DATA_BLOCK DB 63
VERSION : 0.1


  STRUCT
   Messwert : REAL  := 1.000000e+000;
   Messwert1 : REAL  := 1.500000e+000;
   Messwert2 : REAL  := 2.000000e+000;
   Messwert3 : REAL  := 2.500000e+000;
   Messwert4 : REAL  := 3.000000e+000;
   Messwert5 : REAL  := 3.500000e+000;
   Messwert6 : REAL  := 4.000000e+000;
   Messwert7 : REAL  := 4.500000e+000;
   Messwert8 : REAL  := 5.000000e+000;
   Messwert9 : REAL  := 5.500000e+000;
   Messwert10 : REAL  := 6.000000e+000;
   Messwert11 : REAL  := 6.500000e+000;
   Messwert12 : REAL  := 7.000000e+000;
   Messwert13 : REAL  := 7.500000e+000;
   Messwert14 : REAL  := 8.000000e+000;
   Messwert15 : REAL  := 8.500000e+000;
   Messwert16 : REAL  := 9.000000e+000;
   Messwert17 : REAL  := 9.500000e+000;
   Messwert18 : REAL  := 5.000000e-001;
   Messwert19 : REAL  := 1.000000e-001;
   Messwert20 : REAL  := 1.500000e-001;
   Messwert21 : REAL  := 2.500000e-001;
   Messwert22 : REAL  := 3.500000e-001;
   Messwert23 : REAL  := 4.500000e-001;
   Messwert24 : REAL  := 5.500000e-001;
   Messwert25 : REAL  := 6.500000e-001;
   Messwert26 : REAL  := 7.500000e-001;
   Messwert27 : REAL  := 8.500000e-001;
   Messwert28 : REAL  := 9.500000e-001;
   Messwert29 : REAL  := 2.000000e-001;
  END_STRUCT ;
BEGIN
   Messwert := 1.000000e+000;
   Messwert1 := 1.500000e+000;
   Messwert2 := 2.000000e+000;
   Messwert3 := 2.500000e+000;
   Messwert4 := 3.000000e+000;
   Messwert5 := 3.500000e+000;
   Messwert6 := 4.000000e+000;
   Messwert7 := 4.500000e+000;
   Messwert8 := 5.000000e+000;
   Messwert9 := 5.500000e+000;
   Messwert10 := 6.000000e+000;
   Messwert11 := 6.500000e+000;
   Messwert12 := 7.000000e+000;
   Messwert13 := 7.500000e+000;
   Messwert14 := 8.000000e+000;
   Messwert15 := 8.500000e+000;
   Messwert16 := 9.000000e+000;
   Messwert17 := 9.500000e+000;
   Messwert18 := 5.000000e-001;
   Messwert19 := 1.000000e-001;
   Messwert20 := 1.500000e-001;
   Messwert21 := 2.500000e-001;
   Messwert22 := 3.500000e-001;
   Messwert23 := 4.500000e-001;
   Messwert24 := 5.500000e-001;
   Messwert25 := 6.500000e-001;
   Messwert26 := 7.500000e-001;
   Messwert27 := 8.500000e-001;
   Messwert28 := 9.500000e-001;
   Messwert29 := 2.000000e-001;
END_DATA_BLOCK

